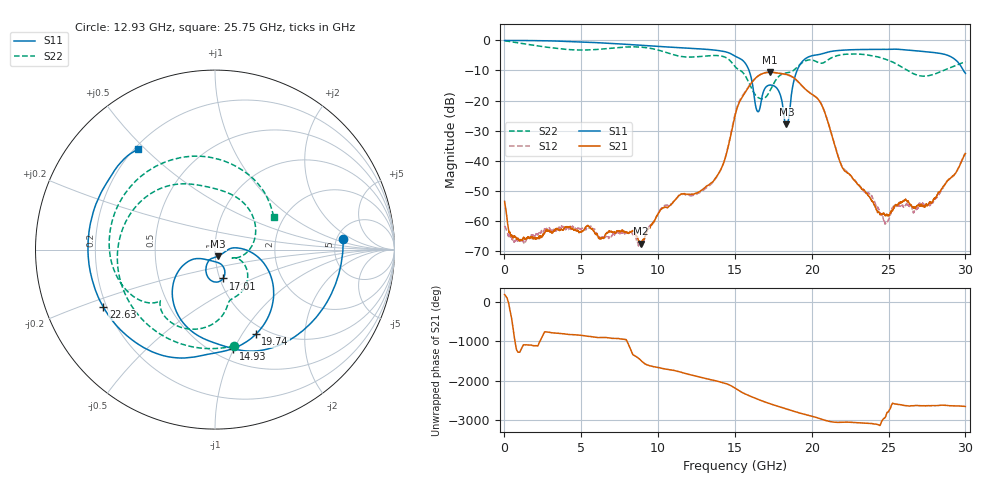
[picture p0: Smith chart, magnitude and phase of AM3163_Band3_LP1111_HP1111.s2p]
!Agilent Technologies,E8364B,MY43040894,A.07.50.67
!Agilent E8364B: A.07.50.67
!Date: Thursday, August 20, 2020 11:06:44
!Correction: S11(Full 2 Port(1,2))
!S21(Full 2 Port(1,2))
!S12(Full 2 Port(1,2))
!S22(Full 2 Port(1,2))
!S2P File: Measurements: S11, S21, S12, S22:
# Hz S  dB  R 50
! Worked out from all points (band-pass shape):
!   3201 points, 10 MHz to 30 GHz, reference 50 ohm
!   highest |S21| = -10.61 dB at 17.28 GHz (marker M1); lowest = -67.6 dB at 8.895 GHz (marker M2)
!   |S21| within 3 dB of the highest: 16.16 GHz to 19.09 GHz (2.938 GHz wide, 16.7 % of centre)
!   lowest |S11| = -27.9 dB at 18.35 GHz (marker M3), VSWR 1.08, Z = 51.5 - j3.78 ohm
!   |S11| at or under -10 dB: 15.92 GHz to 19.04 GHz (3.125 GHz wide, 17.9 % of centre); 29.86945 GHz to end of sweep
!   |S22| runs from -19.4 to -0.1 dB; largest |S21 - S12| = 0.0057
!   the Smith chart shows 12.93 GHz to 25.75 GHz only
!   S11 on the Smith chart (normalised r, x): 12.93 GHz: 5.73, +1.35; 14.93 GHz: 0.62, -0.99; 17.01 GHz: 1.04, -0.34; 19.74 GHz: 0.88, -1.15; 22.63 GHz: 0.19, -0.23; 25.75 GHz: 0.21, +0.48
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1e7  -0.03 -2.1  -53.50 176.1  -61.63 -111.6  -0.14 -5.0
1.256459e9  -0.05 -33.0  -65.43 -12.5  -67.16 -15.3  -1.12 -81.9
2.680984e9  -0.14 -70.0  -63.34 -44.4  -62.90 -57.5  -2.21 -161.8
5.014581e9  -0.53 -128.3  -63.57 -133.4  -62.54 -134.0  -3.20 77.4
6.785866e9  -0.98 -171.7  -63.44 163.0  -65.79 158.3  -2.66 -18.2
8.894538e9  -1.63 133.8  -67.57 -51.6  -68.09 -40.5  -2.25 -136.3
1.000979e10  -1.99 102.1  -57.52 134.5  -57.45 135.2  -3.22 153.0
1.168736e10  -2.51 49.0  -50.91 -6.1  -51.04 -5.6  -5.47 20.8
1.293382e10  -2.89 4.6  -49.39 -125.3  -49.80 -125.2  -5.25 -78.8
1.407718e10  -3.49 -40.5  -42.99 127.8  -42.99 132.8  -5.17 -167.7
1.493002e10  -5.01 -79.5  -26.66 -6.6  -26.18 -5.0  -8.26 109.4
1.5005e10  -5.23 -82.7  -25.01 -25.2  -24.53 -23.9  -8.71 102.8
1.646701e10  -23.59 -112.5  -11.99 56.4  -11.97 56.1  -18.85 -24.6
1.701058e10  -15.55 -74.3  -10.73 -23.2  -10.66 -23.3  -18.85 -23.4
1.728237e10  -14.84 -86.0  -10.61 -59.7  -10.53 -60.1  -16.70 -22.0
1.835076e10  -27.92 -65.6  -11.31 169.9  -11.42 169.5  -10.82 -68.1
1.97378e10  -5.61 -64.3  -16.91 13.1  -16.89 14.2  -6.57 -110.7
2.000958e10  -5.11 -76.9  -17.92 -13.8  -17.85 -12.7  -6.52 -123.0
2.263371e10  -3.10 -152.8  -45.56 -167.4  -45.68 -168.1  -4.52 164.9
2.500479e10  -2.99 148.5  -58.11 113.3  -59.62 53.3  -6.65 69.5
2.575454e10  -3.03 127.4  -53.91 -83.5  -55.08 58.0  -8.56 28.9
3e10  -10.93 -18.0  -37.62 -127.9  -37.43 -127.9  -7.12 131.7
